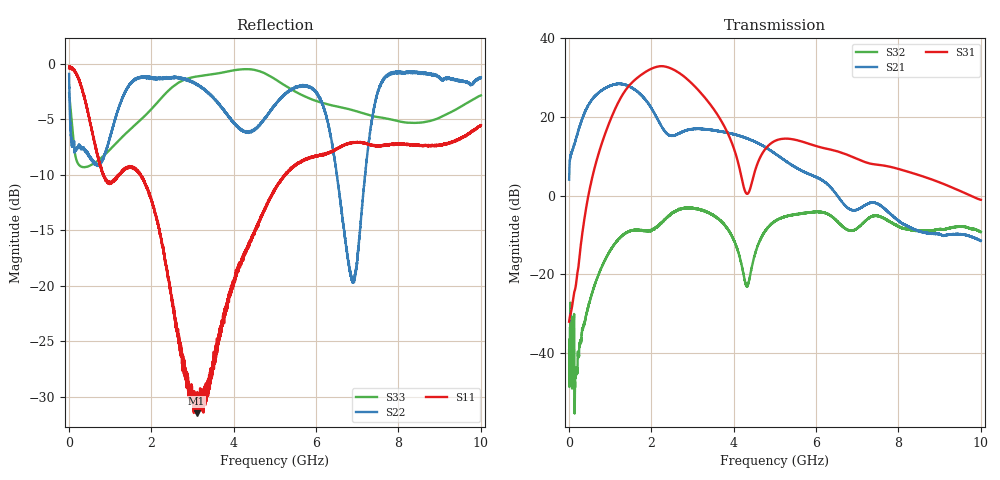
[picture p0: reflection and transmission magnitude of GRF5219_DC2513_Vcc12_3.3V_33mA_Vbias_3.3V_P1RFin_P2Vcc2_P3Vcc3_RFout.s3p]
!Keysight Technologies,N5245B,MY56052315,A.20.20.05
!Date: Friday, August 21, 2026 15:40:22
!Correction: S11(C  3-Port  )
!S12(C  3-Port  )
!S13(C  3-Port  )
!S21(C  3-Port  )
!S22(C  3-Port  )
!S23(C  3-Port  )
!S31(C  3-Port  )
!S32(C  3-Port  )
!S33(C  3-Port  )
!S3P File: Measurements: <S11,S12,S13>,
!<S21,S22,S23>,
!<S31,S32,S33>:
# Hz S  dB  R 50
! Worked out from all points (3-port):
!   9991 points, 10 MHz to 10 GHz, reference 50 ohm
!   strongest paths, dB at 10 MHz, 2.507 GHz, 5.005 GHz, 7.503 GHz, 10 GHz:
!     S31: -32.1, 32.3, 13.9, 7.9, -1.1
!     S21: 4.1, 15.2, 10.7, -2.1, -11.5
!     S32: -39.4, -4.5, -6.5, -5.2, -9.3
!   lowest |S11| = -31.5 dB at 3.103 GHz (marker M1), VSWR 1.05, Z = 52.6 - j0.786 ohm
!   |S11| at or under -10 dB: 842.7 MHz to 1.213 GHz (369.9 MHz wide, 36 % of centre); 1.217136 GHz to 1.22291 GHz (5.775 MHz wide, 0.473 % of centre); 1.745 GHz to 5.243 GHz (3.498 GHz wide, 100 % of centre)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
1e7  -0.38 -1.8  -51.15 50.2  -54.65 165.6
     4.07 81.1  -0.91 -40.8  -53.53 -144.0
     -32.08 -168.1  -39.43 6.9  -2.67 -54.4
8.91e8  -10.42 -93.5  -38.70 78.3  -63.10 70.2
        27.38 -16.6  -7.99 -167.5  -40.42 -117.7
        15.97 -42.7  -16.22 -41.4  -8.14 -152.7
1.407e9  -9.33 -117.6  -37.63 82.2  -59.74 68.9
         28.07 -81.7  -2.31 -166.8  -34.17 177.8
         27.25 -122.5  -9.48 -101.9  -6.21 -151.7
1.895e9  -11.10 -172.5  -34.50 84.9  -61.54 68.9
         23.99 -137.2  -1.19 166.7  -32.56 133.4
         31.69 160.5  -8.99 -138.6  -4.52 -153.3
2.355e9  -17.95 132.8  -33.24 82.4  -59.04 77.3
         16.12 -151.3  -1.25 144.6  -30.69 108.0
         32.83 89.2  -5.87 -150.7  -2.66 -159.1
2.704e9  -25.17 82.1  -32.43 87.0  -57.27 79.0
         15.94 -137.2  -1.29 134.8  -29.48 83.7
         31.06 40.5  -3.48 178.7  -1.62 -168.4
3.103e9  -31.51 -16.3  -31.01 90.2  -59.12 64.3
         17.03 -152.3  -1.80 132.7  -29.53 55.1
         27.33 -7.7  -3.33 142.7  -1.15 -179.7
3.877e9  -21.19 -168.2  -27.69 86.5  -57.95 69.9
         15.90 169.8  -4.77 129.5  -32.85 8.6
         15.47 -80.7  -8.85 81.1  -0.68 163.6
5.005e9  -11.39 170.0  -26.72 70.1  -54.83 113.5
         10.72 110.4  -3.72 119.4  -37.65 59.7
         13.93 -26.5  -6.46 134.6  -1.38 145.8
1e10  -5.53 108.2  -25.10 34.7  -52.04 25.1
      -11.50 57.3  -1.25 86.6  -30.46 -27.5
      -1.05 113.4  -9.30 -50.1  -2.85 82.5
